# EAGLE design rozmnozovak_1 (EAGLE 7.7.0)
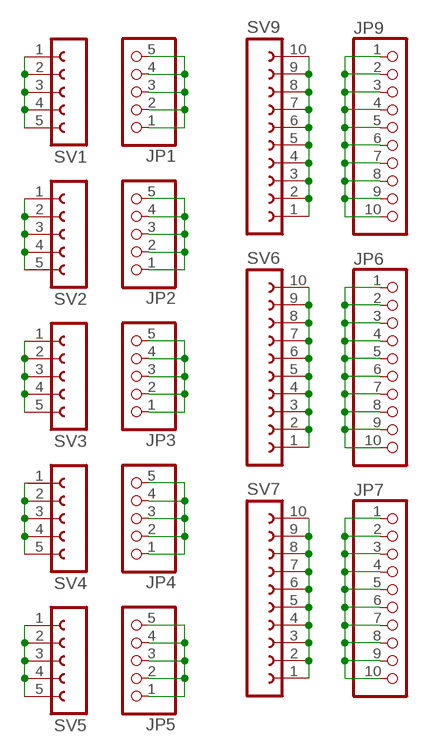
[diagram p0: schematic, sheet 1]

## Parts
JP1  PINHD-1X5  [1X05]
JP2  PINHD-1X5  [1X05]
JP3  PINHD-1X5  [1X05]
JP4  PINHD-1X5  [1X05]
JP5  PINHD-1X5  [1X05]
JP6  PINHD-1X10  [1X10]
JP7  PINHD-1X10  [1X10]
JP9  PINHD-1X10  [1X10]
SV1  FE05-1  [FE05-1]
SV2  FE05-1  [FE05-1]
SV3  FE05-1  [FE05-1]
SV4  FE05-1  [FE05-1]
SV5  FE05-1  [FE05-1]
SV6  FE10-1  [FE10]
SV7  FE10-1  [FE10]
SV9  FE10-1  [FE10]

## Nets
N$1: SV4.1 SV4.2 SV4.3 SV4.4 SV4.5
N$2: SV3.1 SV3.2 SV3.3 SV3.4 SV3.5
N$3: SV2.1 SV2.2 SV2.3 SV2.4 SV2.5
N$4: SV1.1 SV1.2 SV1.3 SV1.4 SV1.5
N$5: JP4.1 JP4.2 JP4.3 JP4.4 JP4.5
N$6: JP3.1 JP3.2 JP3.3 JP3.4 JP3.5
N$7: JP2.1 JP2.2 JP2.3 JP2.4 JP2.5
N$8: JP1.1 JP1.2 JP1.3 JP1.4 JP1.5
N$9: SV6.1 SV6.2 SV6.3 SV6.4 SV6.5 SV6.6 SV6.7 SV6.8 SV6.9 SV6.10
N$10: SV9.1 SV9.2 SV9.3 SV9.4 SV9.5 SV9.6 SV9.7 SV9.8 SV9.9 SV9.10
N$11: JP9.1 JP9.2 JP9.3 JP9.4 JP9.5 JP9.6 JP9.7 JP9.8 JP9.9 JP9.10
N$12: JP6.1 JP6.2 JP6.3 JP6.4 JP6.5 JP6.6 JP6.7 JP6.8 JP6.9 JP6.10
N$13: JP7.1 JP7.2 JP7.3 JP7.4 JP7.5 JP7.6 JP7.7 JP7.8 JP7.9 JP7.10
N$14: SV5.1 SV5.2 SV5.3 SV5.4 SV5.5
N$15: JP5.1 JP5.2 JP5.3 JP5.4 JP5.5
N$16: SV7.1 SV7.2 SV7.3 SV7.4 SV7.5 SV7.6 SV7.7 SV7.8 SV7.9 SV7.10

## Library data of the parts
JP1-JP5 = pinhead:PINHD-1X5: PIN HEADER
JP6 JP7 JP9 = pinhead:PINHD-1X10: PIN HEADER
SV1-SV5 = con-lsta:FE05-1: FEMALE HEADER; OC_FARNELL: unknown; OC_NEWARK: unknown
SV6 SV7 SV9 = con-lsta:FE10-1: FEMALE HEADER; OC_FARNELL: unknown; OC_NEWARK: unknown

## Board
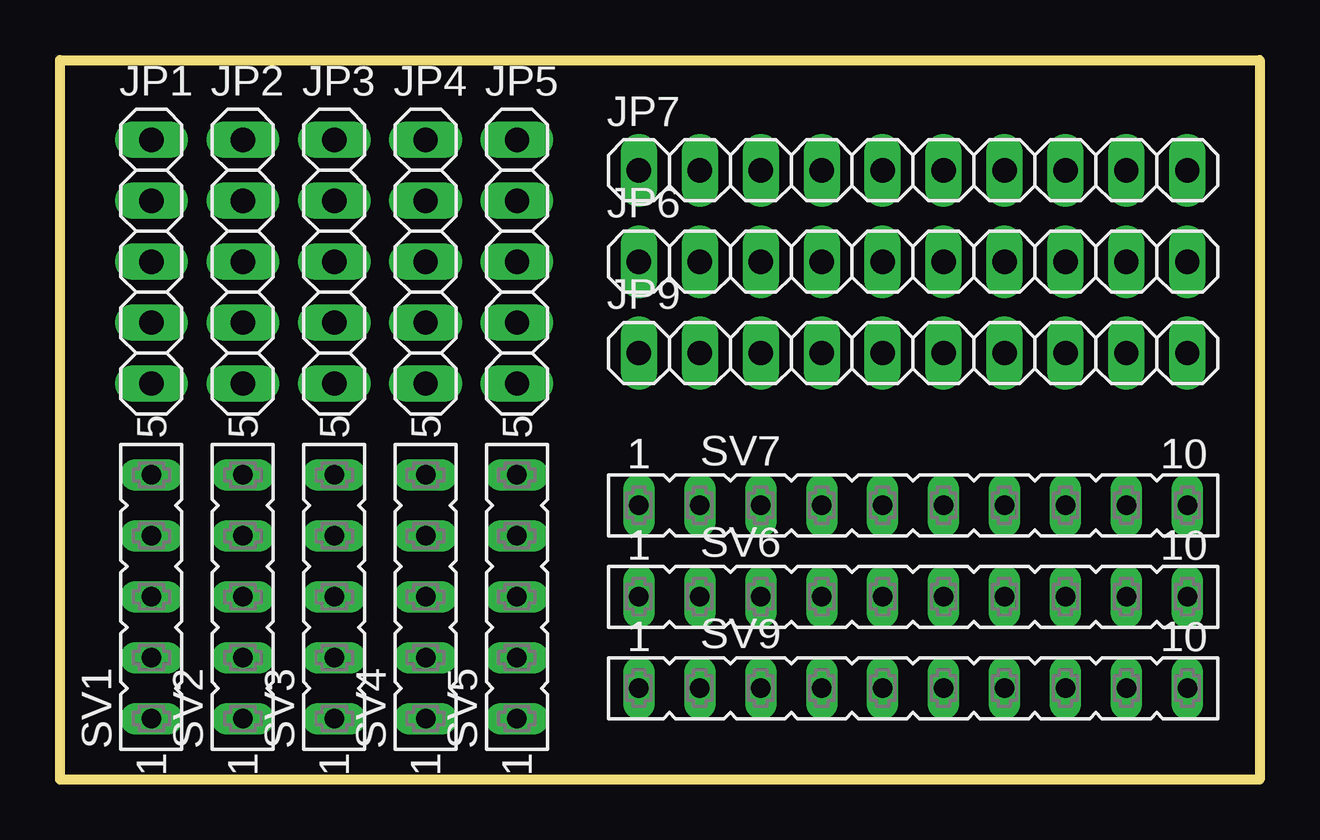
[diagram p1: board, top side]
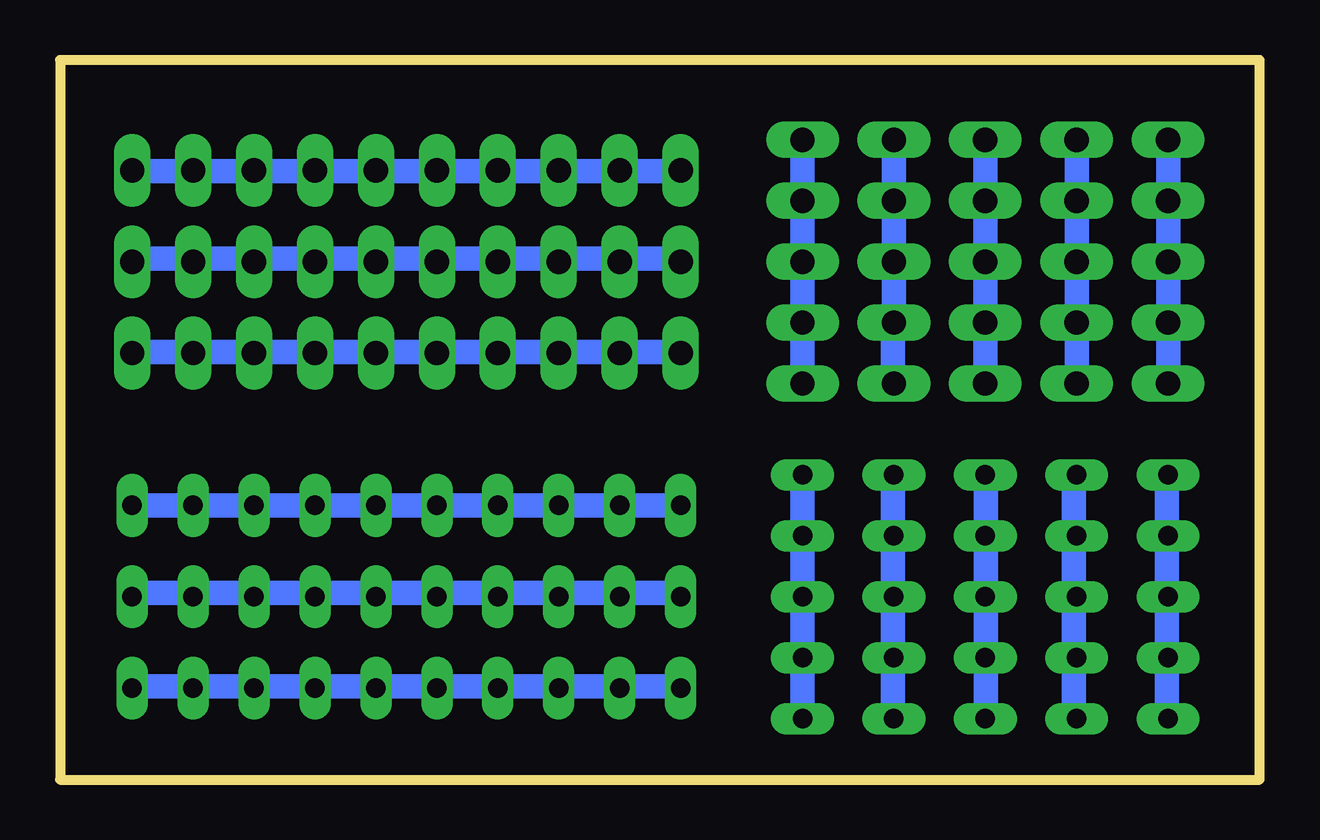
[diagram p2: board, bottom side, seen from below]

Size 50 x 30 mm. Coordinates in mm from the lower left corner, seen from the top.
Outline: 0,0 0,30 50,30 50,0 0,0
Copper layers (1*16): Top 0.035mm / dielectric 1.5mm / Bottom 0.035mm
Design rules "default": minimum track width 10mil, minimum drill 24mil, track to track 8mil, track to pad 8mil, pad to pad 8mil, via to via 8mil, smd to smd 8mil, copper to edge 40mil, drill to drill 8mil, minimum pad ring 10mil, minimum via ring 8mil, stop-mask expansion 4mil, vias tented up to drill 0mil, thermal gap 10mil

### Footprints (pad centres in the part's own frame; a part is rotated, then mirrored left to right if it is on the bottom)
1X05 = drill 1.016 long: 1 -5.08,0; 2 -2.54,0; 3 0,0; 4 2.54,0; 5 5.08,0
1X10 = drill 1.016 long: 1 -11.43,0; 2 -8.89,0; 3 -6.35,0; 4 -3.81,0; 5 -1.27,0; 6 1.27,0; 7 3.81,0; 8 6.35,0; 9 8.89,0; 10 11.43,0
FE05-1 = drill 0.813 long: 1 -5.08,0; 2 -2.54,0; 3 0,0; 4 2.54,0; 5 5.08,0
FE10 = drill 0.813 long: 1 -11.43,0; 2 -8.89,0; 3 -6.35,0; 4 -3.81,0; 5 -1.27,0; 6 1.27,0; 7 3.81,0; 8 6.35,0; 9 8.89,0; 10 11.43,0

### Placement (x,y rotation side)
JP1  3.81,21.59 90 top
JP2  7.62,21.59 90 top
JP3  11.43,21.59 90 top
JP4  15.24,21.59 90 top
JP5  19.05,21.59 90 top
JP6  35.56,21.59 0 top
JP7  35.56,25.4 0 top
JP9  35.56,17.78 0 top
SV1  3.81,7.62 90 top
SV2  7.62,7.62 90 top
SV3  11.43,7.62 90 top
SV4  15.24,7.62 90 top
SV5  19.05,7.62 90 top
SV6  35.56,7.62 0 top
SV7  35.56,11.43 0 top
SV9  35.56,3.81 0 top

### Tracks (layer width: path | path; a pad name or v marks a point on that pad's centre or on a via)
N$1
  Bottom 0.254: 15.29,2.74 SV4.1 | 15.29,5.03 SV4.2 15.29,5.26 | 15.29,7.77 SV4.3 15.29,7.54 | 15.29,10.06 SV4.4 15.29,10.29 | 15.29,12.57 SV4.5
  Bottom 1.016: 15.29,5.03 15.29,2.74 | 15.29,10.06 15.29,7.77 | 15.29,10.29 15.29,12.57 | 15.29,7.54 15.29,5.26
N$2
  Bottom 0.254: 11.4,2.74 SV3.1 | 11.4,5.03 SV3.2 11.4,5.26 | 11.4,7.77 SV3.3 11.4,7.54 | 11.4,10.06 SV3.4 11.4,10.29 | 11.4,12.57 SV3.5
  Bottom 1.016: 11.4,5.03 11.4,2.74 | 11.4,10.06 11.4,7.77 | 11.4,10.29 11.4,12.57 | 11.4,7.54 11.4,5.26
N$3
  Bottom 0.254: 7.75,2.74 SV2.1 | 7.75,5.03 SV2.2 7.75,5.26 | 7.75,7.77 SV2.3 7.75,7.54 | 7.75,10.06 SV2.4 7.75,10.29 | 7.75,12.57 SV2.5
  Bottom 1.016: 7.75,5.03 7.75,2.74 | 7.75,10.06 7.75,7.77 | 7.75,10.29 7.75,12.57 | 7.75,7.54 7.75,5.26
N$4
  Bottom 0.254: 3.86,2.74 SV1.1 | 3.86,5.03 SV1.2 3.86,5.26 | 3.86,7.77 SV1.3 3.86,7.54 | 3.86,10.06 SV1.4 3.86,10.29 | 3.86,12.57 SV1.5
  Bottom 1.016: 3.86,5.03 3.86,2.74 | 3.86,10.06 3.86,7.77 | 3.86,10.29 3.86,12.57 | 3.86,7.54 3.86,5.26
N$5
  Bottom 0.254: 15.29,16.69 JP4.1 | 15.29,18.75 JP4.2
  Bottom 1.016: JP4.5 JP4.4 JP4.3 JP4.2 | 15.29,18.75 15.29,16.69
N$6
  Bottom 1.016: JP3.5 JP3.4 JP3.3 JP3.2 JP3.1
N$7
  Bottom 1.016: JP2.5 JP2.4 JP2.3 JP2.2 JP2.1
N$8
  Bottom 1.016: JP1.5 JP1.4 JP1.3 JP1.2 JP1.1
N$9
  Bottom 0.254: 39.45,7.77 SV6.7 39.22,7.77 | 41.73,7.77 SV6.8 41.96,7.77 | 44.25,7.77 SV6.9 44.48,7.77 | 46.99,7.77 SV6.10 | 34.42,7.77 SV6.5 34.19,7.77 | 36.7,7.77 SV6.6 36.93,7.77 | 24.13,7.77 SV6.1 | 26.64,7.77 SV6.2 | 29.39,7.77 SV6.3 | 31.67,7.77 SV6.4
  Bottom 1.016: 41.73,7.77 39.45,7.77 | 41.96,7.77 44.25,7.77 | 44.48,7.77 46.99,7.77 | 36.7,7.77 34.42,7.77 | 26.64,7.77 24.13,7.77 | 31.67,7.77 29.39,7.77 | SV6.2 26.87,7.77 29.16,7.77 SV6.3 | 34.19,7.77 31.9,7.77 SV6.4 | 36.93,7.77 39.22,7.77
N$10
  Bottom 0.254: 39.45,3.89 SV9.7 39.22,3.89 | 41.73,3.89 SV9.8 | 44.25,3.89 SV9.9 44.48,3.89 | 46.99,3.89 SV9.10 | 34.42,3.89 SV9.5 34.19,3.89 | 36.7,3.89 SV9.6 36.93,3.89 | 24.13,3.89 SV9.1 | 26.64,3.89 SV9.2 26.87,3.89 | 29.39,3.89 SV9.3 29.16,3.89 | 31.67,3.89 SV9.4 31.9,3.89
  Bottom 1.016: 41.73,3.89 39.45,3.89 | 44.25,3.89 41.96,3.89 SV9.8 | 44.48,3.89 46.99,3.89 | 36.7,3.89 34.42,3.89 | 26.64,3.89 24.13,3.89 | 31.67,3.89 29.39,3.89 | 29.16,3.89 26.87,3.89 | 31.9,3.89 34.19,3.89 | 36.93,3.89 39.22,3.89
N$11
  Bottom 0.254: 41.96,17.83 JP9.8 41.73,17.83 | 44.25,17.83 JP9.9 44.48,17.83 | 46.99,17.83 JP9.10 | 36.93,17.83 JP9.6 | 39.22,17.83 JP9.7 39.45,17.83 | 31.9,17.83 JP9.4 31.67,17.83 | 34.19,17.83 JP9.5 34.42,17.83 | 24.13,17.83 JP9.1 | 26.64,17.83 JP9.2 26.87,17.83 | 29.16,17.83 JP9.3 29.39,17.83
  Bottom 1.016: 44.25,17.83 41.96,17.83 | 44.48,17.83 46.99,17.83 | 39.22,17.83 36.93,17.83 | 34.19,17.83 31.9,17.83 | 26.64,17.83 24.13,17.83 | 26.87,17.83 29.16,17.83 | 29.39,17.83 31.67,17.83 | 34.42,17.83 36.7,17.83 JP9.6 | 39.45,17.83 41.73,17.83
N$12
  Bottom 0.254: 41.96,21.72 JP6.8 41.73,21.72 | 44.25,21.72 JP6.9 44.48,21.72 | 46.99,21.72 JP6.10 | 36.93,21.72 JP6.6 36.7,21.72 | 39.22,21.72 JP6.7 39.45,21.72 | 31.9,21.72 JP6.4 31.67,21.72 | 34.19,21.72 JP6.5 34.42,21.72 | 24.13,21.72 JP6.1 | 26.64,21.72 JP6.2 26.87,21.72 | 29.16,21.72 JP6.3 29.39,21.72
  Bottom 1.016: 44.25,21.72 41.96,21.72 | 44.48,21.72 46.99,21.72 | 39.22,21.72 36.93,21.72 | 34.19,21.72 31.9,21.72 | 26.64,21.72 24.13,21.72 | 26.87,21.72 29.16,21.72 | 29.39,21.72 31.67,21.72 | 34.42,21.72 36.7,21.72 | 39.45,21.72 41.73,21.72
N$13
  Bottom 0.254: 41.96,25.38 JP7.8 41.73,25.38 | 44.25,25.38 JP7.9 44.48,25.38 | 46.99,25.38 JP7.10 | 36.93,25.38 JP7.6 36.7,25.38 | 31.9,25.38 JP7.4 31.67,25.38 | 34.19,25.38 JP7.5 34.42,25.38 | 24.13,25.38 JP7.1 | 26.64,25.38 JP7.2 26.87,25.38 | 29.16,25.38 JP7.3 29.39,25.38 | 39.45,25.38 JP7.7
  Bottom 1.016: 44.25,25.38 41.96,25.38 | 44.48,25.38 46.99,25.38 | 36.93,25.38 39.22,25.38 JP7.7 | 34.19,25.38 31.9,25.38 | 26.64,25.38 24.13,25.38 | 26.87,25.38 29.16,25.38 | 29.39,25.38 31.67,25.38 | 34.42,25.38 36.7,25.38 | 39.45,25.38 41.73,25.38
N$14
  Bottom 1.016: SV5.5 SV5.4 SV5.3 SV5.2 SV5.1
N$15
  Bottom 1.016: JP5.5 JP5.4 JP5.3 JP5.2 JP5.1
N$16
  Bottom 1.016: SV7.10 SV7.9 SV7.8 SV7.7 SV7.6 SV7.5 SV7.4 SV7.3 SV7.2 SV7.1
